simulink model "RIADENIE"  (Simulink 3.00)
settings: Solver=ode45  SolverMode=SingleTasking  StartTime=0.0  StopTime=1.5  FixedStep=0.00001  MaxStep=Auto  RelTol=1e-5
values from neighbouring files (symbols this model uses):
  J = 0.0017    [Data.m]
  Km = Tim/(K3*Tw3)    [Regulatory.m]
  Kmt = Timt/(K2*Tw2)    [Regulatory.m]
  Kpp = T1/(K1*Tw1)    [Regulatory.m]
  kr = Lm/Lr    (= 0.963591022444)    [Data.m]
  Lm = .5796    (= 0.5796)    [Data.m]
  Ls1 = Ls-Lm^2/Lr    (= 0.0430026433915)    [Data.m]
  p = 1    [Data.m]
  R1 = Rs+kr^2*Rr    (= 11.0434783366)    [Data.m]
  T1 = Ls1/R1    (= 0.00389394012293)    [Data.m]
  Tim = (T1*R1)/(Kpp)    [Regulatory.m]
  Timt = Tr    [Regulatory.m]
  Tip = T1    [Regulatory.m]
  Tr = Lr/Rr    (= 0.162567567568)    [Data.m]
  Tvz = 0.001    [Regulatory.m]
undefined symbols (not defined in the file or in its folder): km
libraries: simulink_extras x1

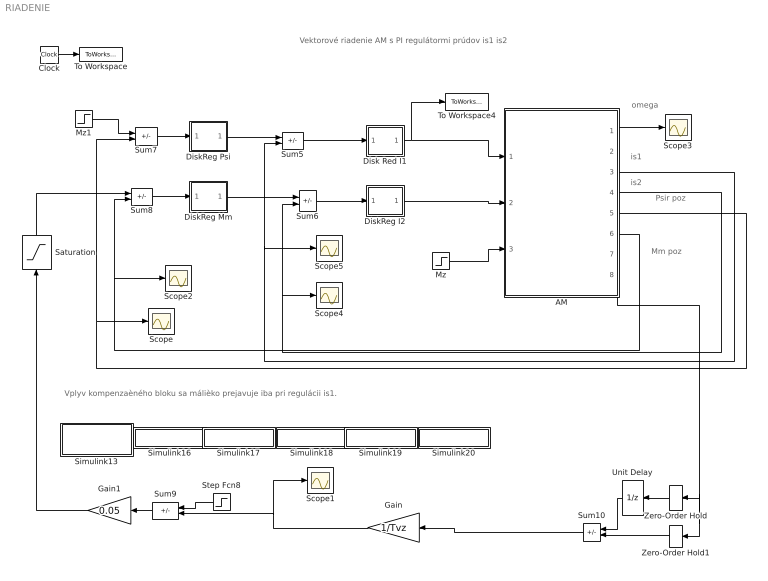
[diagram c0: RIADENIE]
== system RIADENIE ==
  note: omega
  note: Psir poz
  note: Mm poz
  note: is1
  note: is2
  note: Vektorové riadenie AM s PI regulátormi prúdov is1 is2
  note: Vplyv kompenzaèného bloku sa málièko prejavuje iba pri regulácii is1.
  AM : Subsystem
  Clock : Clock
  Disk Red I1 : Subsystem
  DiskReg I2 : Subsystem
  DiskReg Mm : Subsystem
  DiskReg Psi : Subsystem
  Gain : Gain  Orientation=left  Gain=1/Tvz  SaturateOnIntegerOverflow=on
  Gain1 : Gain  Orientation=left  Gain=0.05  SaturateOnIntegerOverflow=on
  Mz : Step  Description=Mz  Time=0  Before=0  After=0  SampleTime=0
  Mz1 : Step  Description=Mz  Time=0  Before=0  After=1  SampleTime=0
  Saturation : Saturate  Orientation=up  UpperLimit=135  LowerLimit=-135
  Scope{,1..5} (6 alike) : Scope
  Simulink13 : Subsystem
  Simulink16 : Subsystem
  Simulink17 : Subsystem
  Simulink18 : Subsystem
  Simulink19 : Subsystem
  Simulink20 : Subsystem
  Step Fcn8 : Step  Orientation=left  Time=0  Before=0  After=100  SampleTime=0
  Sum10 : Sum  Orientation=left  Inputs=-+  SaturateOnIntegerOverflow=on
  Sum{5..8} (4 alike) : Sum  Inputs=+-  SaturateOnIntegerOverflow=on
  Sum9 : Sum  Orientation=left  Inputs=+-  SaturateOnIntegerOverflow=on
  To Workspace : ToWorkspace  VariableName=t  SampleTime=0  SaveFormat=Matrix
  To Workspace4 : ToWorkspace  VariableName=u  SampleTime=0  SaveFormat=Matrix
  Unit Delay : UnitDelay  Orientation=left  X0=0  SampleTime=Tvz
  Zero-Order Hold : ZeroOrderHold  Orientation=left  SampleTime=Tvz
  Zero-Order Hold1 : ZeroOrderHold  Orientation=left  SampleTime=Tvz
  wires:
  Clock/1 -> To Workspace/1
  Sum5/1 -> Disk Red I1/1(In1)
  Disk Red I1/1(Out1) -> AM/1(us1), To Workspace4/1
  Sum6/1 -> DiskReg I2/1(In1)
  DiskReg I2/1(Out1) -> AM/2(us2)
  Sum7/1 -> DiskReg Psi/1(In1)
  Sum8/1 -> DiskReg Mm/1(In1)
  Mz/1 -> AM/3(Mz)
  Step Fcn8/1 -> Sum9/1
  DiskReg Psi/1(Out1) -> Sum5/1
  DiskReg Mm/1(Out1) -> Sum6/1
  Gain1/1 -> Saturation/1
  AM/5(PsirPoz) -> Sum7/2, Scope/1
  AM/4(is2) -> Sum6/2, Scope4/1
  AM/3(is1) -> Sum5/2, Scope5/1
  Saturation/1 -> Sum8/1
  Sum9/1 -> Gain1/1
  Mz1/1 -> Sum7/1
  AM/6(MmPoz) -> Sum8/2, Scope2/1
  Zero-Order Hold1/1 -> Sum10/2
  Unit Delay/1 -> Sum10/1
  Zero-Order Hold/1 -> Unit Delay/1
  AM/1(omega) -> Scope3/1
  Gain/1 -> Scope1/1, Sum9/2
  Sum10/1 -> Gain/1
  AM/8(Theta) -> Zero-Order Hold/1, Zero-Order Hold1/1

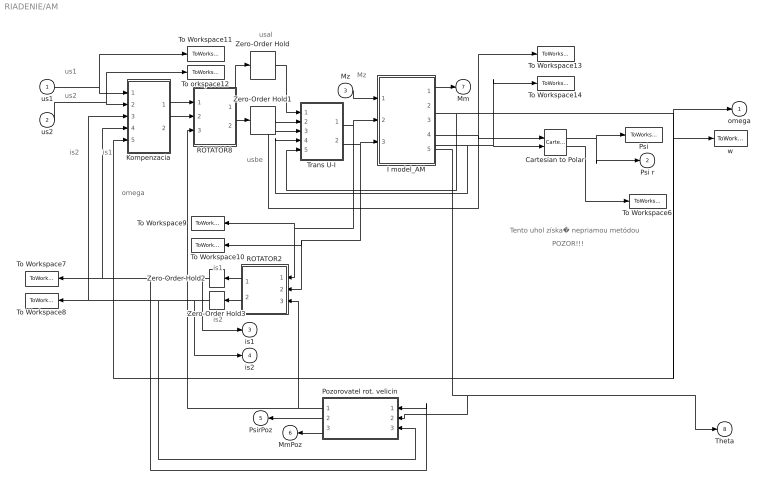
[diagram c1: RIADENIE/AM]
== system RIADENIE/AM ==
  note: is2
  note: is1
  note: omega
  note: us2
  note: us1
  note: Mz
  note: is1
  note: is2
  note: POZOR!!!
  note: Tento uhol získa� nepriamou metódou
  note: usal
  note: usbe
  us1 : Inport  Port=1  PortWidth=-1  SampleTime=-1  DataType=auto
  us2 : Inport  Port=2  PortWidth=-1  SampleTime=-1  DataType=auto
  Mz : Inport  Port=3  PortWidth=-1  SampleTime=-1  DataType=auto
  Cartesian to Polar : simulink_extras/Transformations/Cartesian to Polar
  I model_AM : Subsystem
  Kompenzacia : Subsystem
  Pozorovatel rot. velicin : Subsystem  Orientation=left
  Psi : ToWorkspace  VariableName=Psi  SampleTime=0  SaveFormat=Matrix
  ROTATOR2 : Subsystem  Orientation=left
  ROTATOR8 : Subsystem
  To Workspace10 : ToWorkspace  VariableName=isb  SampleTime=0  SaveFormat=Matrix
  To Workspace11 : ToWorkspace  VariableName=us1  SampleTime=0  SaveFormat=Matrix
  To Workspace13 : ToWorkspace  VariableName=psiral  SampleTime=0  SaveFormat=Matrix
  To Workspace14 : ToWorkspace  VariableName=psirbe  SampleTime=0  SaveFormat=Matrix
  To Workspace6 : ToWorkspace  VariableName=theta  SampleTime=0  SaveFormat=Matrix
  To Workspace7 : ToWorkspace  VariableName=is1  SampleTime=0  SaveFormat=Matrix
  To Workspace8 : ToWorkspace  VariableName=is2  SampleTime=0  SaveFormat=Matrix
  To Workspace9 : ToWorkspace  VariableName=isal  SampleTime=0  SaveFormat=Matrix
  To orkspace12 : ToWorkspace  VariableName=us2  SampleTime=0  SaveFormat=Matrix
  Trans U-I : Subsystem
  Zero-Order Hold : ZeroOrderHold  SampleTime=Tvz
  Zero-Order Hold1 : ZeroOrderHold  SampleTime=Tvz
  Zero-Order Hold2 : ZeroOrderHold  Orientation=left  SampleTime=Tvz
  Zero-Order Hold3 : ZeroOrderHold  Orientation=left  SampleTime=Tvz
  w : ToWorkspace  VariableName=omega  SampleTime=0  SaveFormat=Matrix
  omega : Outport  Port=1  InitialOutput=0
  Psi r : Outport  Port=2  InitialOutput=0
  is1 : Outport  Port=3  InitialOutput=0
  is2 : Outport  Port=4  InitialOutput=0
  PsirPoz : Outport  Orientation=left  Port=5  InitialOutput=0
  MmPoz : Outport  Orientation=left  Port=6  InitialOutput=0
  Mm : Outport  Port=7  InitialOutput=0
  Theta : Outport  Port=8  InitialOutput=0
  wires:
  Kompenzacia/2(Outport2) -> ROTATOR8/2(in_2)
  Kompenzacia/1(Outport1) -> ROTATOR8/1(in_1)
  Trans U-I/2(out_2) -> I model_AM/3(isbe), To Workspace10/1, ROTATOR2/2(in_2)
  Mz/1 -> I model_AM/1(Mz)
  Trans U-I/1(out_1) -> I model_AM/2(isal), To Workspace9/1, ROTATOR2/1(in_1)
  us1/1 -> Kompenzacia/1(in_1), To Workspace11/1
  us2/1 -> Kompenzacia/2(in_2), To orkspace12/1
  Pozorovatel rot. velicin/1(ThetaPoz) -> ROTATOR8/3(in_3), ROTATOR2/3(in_3)
  Pozorovatel rot. velicin/2(PsirPoz) -> PsirPoz/1
  Pozorovatel rot. velicin/3(MmPoz) -> MmPoz/1
  Cartesian to Polar/1 -> Psi/1, Psi r/1
  Cartesian to Polar/2 -> To Workspace6/1
  I model_AM/1(Mm) -> Mm/1
  I model_AM/3(Psir_al) -> Cartesian to Polar/1, To Workspace13/1, Trans U-I/3(in_6)
  I model_AM/4(Psir_be) -> Cartesian to Polar/2, To Workspace14/1, Trans U-I/4(in_4)
  I model_AM/2(omega) -> omega/1, w/1, Kompenzacia/5(in_5), Trans U-I/5(in_8)
  I model_AM/5(Theta) -> Theta/1, Pozorovatel rot. velicin/2(theta)
  ROTATOR8/2(out_2) -> Zero-Order Hold1/1
  Zero-Order Hold1/1 -> Trans U-I/2(in_2)
  ROTATOR8/1(out_1) -> Zero-Order Hold/1
  Zero-Order Hold/1 -> Trans U-I/1(in_1)
  ROTATOR2/1(out_1) -> Zero-Order Hold2/1
  Zero-Order Hold2/1 -> is1/1, Kompenzacia/4(in_6), To Workspace7/1, Pozorovatel rot. velicin/1(Is1)
  ROTATOR2/2(out_2) -> Zero-Order Hold3/1
  Zero-Order Hold3/1 -> is2/1, Kompenzacia/3(in_3), To Workspace8/1, Pozorovatel rot. velicin/3(Is2)

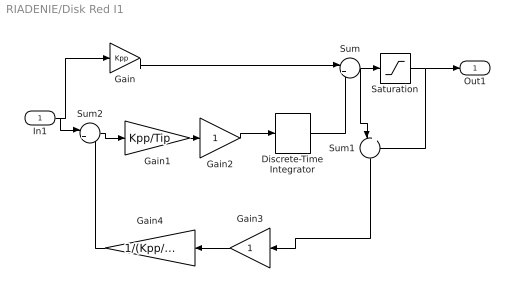
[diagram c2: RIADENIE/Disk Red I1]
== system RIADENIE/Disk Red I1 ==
  In1 : Inport  Port=1  PortWidth=-1  SampleTime=-1  DataType=auto
  Discrete-Time Integrator : DiscreteIntegrator  IntegratorMethod=ForwardEuler  ExternalReset=none  InitialConditionSource=internal  InitialCondition=0  LimitOutput=off  UpperSaturationLimit=inf  LowerSaturationLimit=-inf  ShowSaturationPort=off  ShowStatePort=off  SampleTime=Tvz
  Gain : Gain  Gain=Kpp  SaturateOnIntegerOverflow=on
  Gain1 : Gain  Gain=Kpp/Tip  SaturateOnIntegerOverflow=on
  Gain2 : Gain  Gain=1  SaturateOnIntegerOverflow=on
  Gain3 : Gain  Orientation=left  Gain=1  SaturateOnIntegerOverflow=on
  Gain4 : Gain  Orientation=left  Gain=1/(Kpp/Tip)  SaturateOnIntegerOverflow=on
  Saturation : Saturate  UpperLimit=311  LowerLimit=-311
  Sum : Sum  Inputs=|++  SaturateOnIntegerOverflow=on
  Sum1 : Sum  Orientation=down  Inputs=|+-  SaturateOnIntegerOverflow=on
  Sum2 : Sum  Inputs=|+-  SaturateOnIntegerOverflow=on
  Out1 : Outport  Port=1
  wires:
  Gain3/1 -> Gain4/1
  Saturation/1 -> Sum1/2, Out1/1
  Sum/1 -> Sum1/1, Saturation/1
  Discrete-Time Integrator/1 -> Sum/2
  Gain/1 -> Sum/1
  Gain2/1 -> Discrete-Time Integrator/1
  Gain1/1 -> Gain2/1
  Gain4/1 -> Sum2/2
  In1/1 -> Sum2/1, Gain/1
  Sum2/1 -> Gain1/1
  Sum1/1 -> Gain3/1

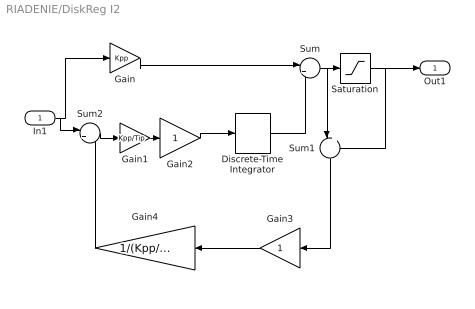
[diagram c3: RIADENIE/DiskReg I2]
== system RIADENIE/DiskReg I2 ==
  In1 : Inport  Port=1  PortWidth=-1  SampleTime=-1  DataType=auto
  Discrete-Time Integrator : DiscreteIntegrator  IntegratorMethod=ForwardEuler  ExternalReset=none  InitialConditionSource=internal  InitialCondition=0  LimitOutput=off  UpperSaturationLimit=inf  LowerSaturationLimit=-inf  ShowSaturationPort=off  ShowStatePort=off  SampleTime=Tvz
  Gain : Gain  Gain=Kpp  SaturateOnIntegerOverflow=on
  Gain1 : Gain  Gain=Kpp/Tip  SaturateOnIntegerOverflow=on
  Gain2 : Gain  Gain=1  SaturateOnIntegerOverflow=on
  Gain3 : Gain  Orientation=left  Gain=1  SaturateOnIntegerOverflow=on
  Gain4 : Gain  Orientation=left  Gain=1/(Kpp/Tip)  SaturateOnIntegerOverflow=on
  Saturation : Saturate  UpperLimit=311  LowerLimit=-311
  Sum : Sum  Inputs=|++  SaturateOnIntegerOverflow=on
  Sum1 : Sum  Orientation=down  Inputs=|+-  SaturateOnIntegerOverflow=on
  Sum2 : Sum  Inputs=|+-  SaturateOnIntegerOverflow=on
  Out1 : Outport  Port=1
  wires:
  Gain1/1 -> Gain2/1
  Gain2/1 -> Discrete-Time Integrator/1
  Gain/1 -> Sum/1
  Discrete-Time Integrator/1 -> Sum/2
  Sum/1 -> Saturation/1, Sum1/1
  Saturation/1 -> Out1/1, Sum1/2
  Sum2/1 -> Gain1/1
  In1/1 -> Gain/1, Sum2/1
  Gain3/1 -> Gain4/1
  Gain4/1 -> Sum2/2
  Sum1/1 -> Gain3/1

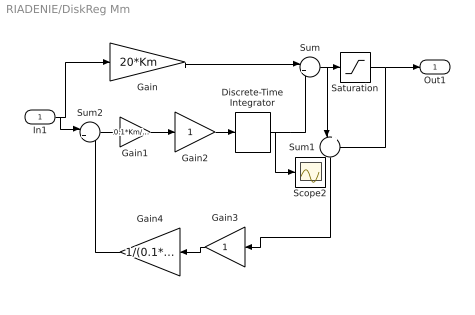
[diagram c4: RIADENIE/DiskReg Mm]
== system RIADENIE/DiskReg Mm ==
  In1 : Inport  Port=1  PortWidth=-1  SampleTime=-1  DataType=auto
  Discrete-Time Integrator : DiscreteIntegrator  IntegratorMethod=ForwardEuler  ExternalReset=none  InitialConditionSource=internal  InitialCondition=0  LimitOutput=off  UpperSaturationLimit=inf  LowerSaturationLimit=-inf  ShowSaturationPort=off  ShowStatePort=off  SampleTime=Tvz
  Gain : Gain  Gain=20*Km  SaturateOnIntegerOverflow=on
  Gain1 : Gain  Gain=0.1*Km/Tim  SaturateOnIntegerOverflow=on
  Gain2 : Gain  Gain=1  SaturateOnIntegerOverflow=on
  Gain3 : Gain  Orientation=left  Gain=1  SaturateOnIntegerOverflow=on
  Gain4 : Gain  Orientation=left  Gain=1/(0.1*Km/Tim)  SaturateOnIntegerOverflow=on
  Saturation : Saturate  UpperLimit=12.28  LowerLimit=-12.28
  Scope2 : Scope
  Sum : Sum  Inputs=|++  SaturateOnIntegerOverflow=on
  Sum1 : Sum  Orientation=down  Inputs=|+-  SaturateOnIntegerOverflow=on
  Sum2 : Sum  Inputs=|+-  SaturateOnIntegerOverflow=on
  Out1 : Outport  Port=1
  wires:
  Gain4/1 -> Sum2/2
  Gain3/1 -> Gain4/1
  In1/1 -> Sum2/1, Gain/1
  Sum2/1 -> Gain1/1
  Saturation/1 -> Sum1/2, Out1/1
  Sum/1 -> Sum1/1, Saturation/1
  Gain/1 -> Sum/1
  Gain2/1 -> Discrete-Time Integrator/1
  Gain1/1 -> Gain2/1
  Sum1/1 -> Gain3/1
  Discrete-Time Integrator/1 -> Sum/2, Scope2/1

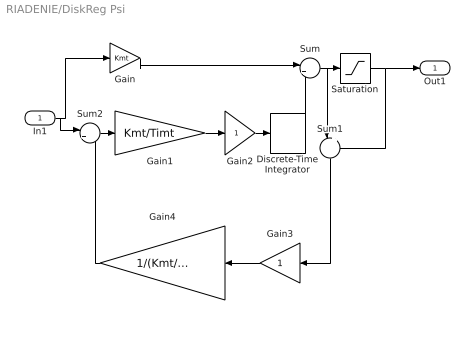
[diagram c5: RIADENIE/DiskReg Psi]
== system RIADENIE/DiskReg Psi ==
  In1 : Inport  Port=1  PortWidth=-1  SampleTime=-1  DataType=auto
  Discrete-Time Integrator : DiscreteIntegrator  IntegratorMethod=ForwardEuler  ExternalReset=none  InitialConditionSource=internal  InitialCondition=0  LimitOutput=off  UpperSaturationLimit=inf  LowerSaturationLimit=-inf  ShowSaturationPort=off  ShowStatePort=off  SampleTime=Tvz
  Gain : Gain  Gain=Kmt  SaturateOnIntegerOverflow=on
  Gain1 : Gain  Gain=Kmt/Timt  SaturateOnIntegerOverflow=on
  Gain2 : Gain  Gain=1  SaturateOnIntegerOverflow=on
  Gain3 : Gain  Orientation=left  Gain=1  SaturateOnIntegerOverflow=on
  Gain4 : Gain  Orientation=left  Gain=1/(Kmt/Timt)  SaturateOnIntegerOverflow=on
  Saturation : Saturate  UpperLimit=12.28  LowerLimit=-12.28
  Sum : Sum  Inputs=|++  SaturateOnIntegerOverflow=on
  Sum1 : Sum  Orientation=down  Inputs=|+-  SaturateOnIntegerOverflow=on
  Sum2 : Sum  Inputs=|+-  SaturateOnIntegerOverflow=on
  Out1 : Outport  Port=1
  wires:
  Gain1/1 -> Gain2/1
  Gain2/1 -> Discrete-Time Integrator/1
  Gain/1 -> Sum/1
  Discrete-Time Integrator/1 -> Sum/2
  Sum/1 -> Saturation/1, Sum1/1
  Saturation/1 -> Out1/1, Sum1/2
  Sum2/1 -> Gain1/1
  In1/1 -> Gain/1, Sum2/1
  Gain3/1 -> Gain4/1
  Gain4/1 -> Sum2/2
  Sum1/1 -> Gain3/1

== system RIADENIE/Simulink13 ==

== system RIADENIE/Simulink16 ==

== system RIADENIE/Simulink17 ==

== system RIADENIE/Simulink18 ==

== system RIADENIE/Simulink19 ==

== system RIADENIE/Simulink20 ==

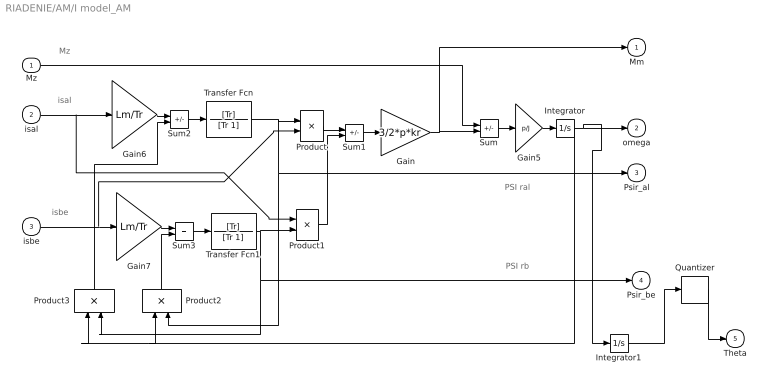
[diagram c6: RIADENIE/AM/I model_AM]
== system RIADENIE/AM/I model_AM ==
  note: isal
  note: PSI ral
  note: isbe
  note: PSI rb
  note: Mz
  Mz : Inport  Port=1  PortWidth=-1  SampleTime=-1  DataType=auto
  isal : Inport  Port=2  PortWidth=-1  SampleTime=-1  DataType=auto
  isbe : Inport  Port=3  PortWidth=-1  SampleTime=-1  DataType=auto
  Gain : Gain  Gain=3/2*p*kr  SaturateOnIntegerOverflow=on
  Gain5 : Gain  Gain=p/J  SaturateOnIntegerOverflow=on
  Gain6 : Gain  Gain=Lm/Tr  SaturateOnIntegerOverflow=on
  Gain7 : Gain  Gain=Lm/Tr  SaturateOnIntegerOverflow=on
  Integrator : Integrator  ExternalReset=none  InitialConditionSource=internal  InitialCondition=0  LimitOutput=off  UpperSaturationLimit=inf  LowerSaturationLimit=-inf  ShowSaturationPort=off  ShowStatePort=off  AbsoluteTolerance=auto
  Integrator1 : Integrator  ExternalReset=none  InitialConditionSource=internal  InitialCondition=0  LimitOutput=off  UpperSaturationLimit=inf  LowerSaturationLimit=-inf  ShowSaturationPort=off  ShowStatePort=off  AbsoluteTolerance=auto
  Product : Product  Inputs=2  SaturateOnIntegerOverflow=on
  Product1 : Product  Inputs=2  SaturateOnIntegerOverflow=on
  Product2 : Product  Orientation=up  Inputs=2  SaturateOnIntegerOverflow=on
  Product3 : Product  Orientation=up  Inputs=2  SaturateOnIntegerOverflow=on
  Quantizer : Quantizer  QuantizationInterval=6.28/4096
  Sum : Sum  Inputs=-+  SaturateOnIntegerOverflow=on
  Sum1 : Sum  Inputs=+-  SaturateOnIntegerOverflow=on
  Sum2 : Sum  Inputs=+-  SaturateOnIntegerOverflow=on
  Sum3 : Sum  Inputs=++  SaturateOnIntegerOverflow=on
  Transfer Fcn : TransferFcn  Numerator=[Tr]  Denominator=[Tr 1]
  Transfer Fcn1 : TransferFcn  Numerator=[Tr]  Denominator=[Tr 1]
  Mm : Outport  Port=1  InitialOutput=0
  omega : Outport  Port=2  InitialOutput=0
  Psir_al : Outport  Port=3  InitialOutput=0
  Psir_be : Outport  Port=4  InitialOutput=0
  Theta : Outport  Port=5  InitialOutput=0
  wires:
  Gain/1 -> Mm/1, Sum/2
  Product1/1 -> Sum1/2
  Mz/1 -> Sum/1
  isbe/1 -> Gain7/1, Product/2
  Product2/1 -> Sum3/2
  Sum3/1 -> Transfer Fcn1/1
  Sum2/1 -> Transfer Fcn/1
  Product/1 -> Sum1/1
  Sum1/1 -> Gain/1
  Sum/1 -> Gain5/1
  Integrator/1 -> Product3/1, Product2/1, omega/1, Integrator1/1
  Transfer Fcn/1 -> Product/1, Product2/2, Psir_al/1
  Gain7/1 -> Sum3/1
  Gain6/1 -> Sum2/1
  Transfer Fcn1/1 -> Product1/2, Product3/2, Psir_be/1
  Product3/1 -> Sum2/2
  isal/1 -> Gain6/1, Product1/1
  Gain5/1 -> Integrator/1
  Integrator1/1 -> Quantizer/1
  Quantizer/1 -> Theta/1

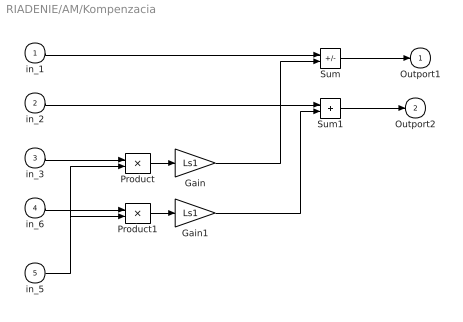
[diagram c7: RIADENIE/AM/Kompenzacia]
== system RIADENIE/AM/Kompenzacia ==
  in_1 : Inport  Port=1  PortWidth=-1  SampleTime=-1  DataType=auto
  in_2 : Inport  Port=2  PortWidth=-1  SampleTime=-1  DataType=auto
  in_3 : Inport  Port=3  PortWidth=-1  SampleTime=-1  DataType=auto
  in_6 : Inport  Port=4  PortWidth=-1  SampleTime=-1  DataType=auto
  in_5 : Inport  Port=5  PortWidth=-1  SampleTime=-1  DataType=auto
  Gain : Gain  Gain=Ls1  SaturateOnIntegerOverflow=on
  Gain1 : Gain  Gain=Ls1  SaturateOnIntegerOverflow=on
  Product : Product  Inputs=2  SaturateOnIntegerOverflow=on
  Product1 : Product  Inputs=2  SaturateOnIntegerOverflow=on
  Sum : Sum  Inputs=+-  SaturateOnIntegerOverflow=on
  Sum1 : Sum  Inputs=++  SaturateOnIntegerOverflow=on
  Outport1 : Outport  Port=1  InitialOutput=0
  Outport2 : Outport  Port=2  InitialOutput=0
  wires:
  Sum1/1 -> Outport2/1
  in_2/1 -> Sum1/1
  Gain1/1 -> Sum1/2
  Product1/1 -> Gain1/1
  in_5/1 -> Product/2, Product1/2
  in_6/1 -> Product1/1
  Sum/1 -> Outport1/1
  Gain/1 -> Sum/2
  in_1/1 -> Sum/1
  Product/1 -> Gain/1
  in_3/1 -> Product/1

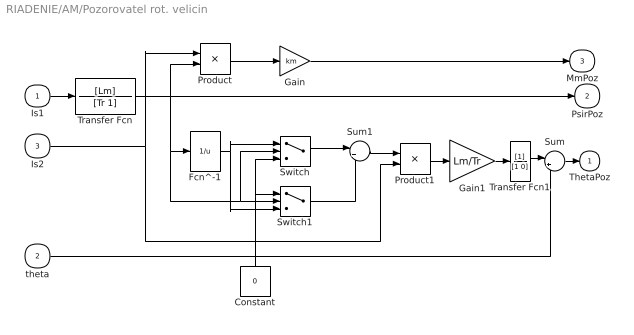
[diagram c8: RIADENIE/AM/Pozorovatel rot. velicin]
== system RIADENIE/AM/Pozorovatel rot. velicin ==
  Is1 : Inport  Port=1  PortWidth=-1  SampleTime=-1  DataType=auto
  theta : Inport  Port=2  PortWidth=-1  SampleTime=-1  DataType=auto
  Is2 : Inport  Port=3  PortWidth=-1  SampleTime=-1  DataType=auto
  Constant : Constant  Orientation=up  Value=0
  Fcn^-1 : Fcn  Expr=1/u
  Gain : Gain  Gain=km  SaturateOnIntegerOverflow=on
  Gain1 : Gain  Gain=Lm/Tr  SaturateOnIntegerOverflow=on
  Product : Product  Inputs=2  SaturateOnIntegerOverflow=on
  Product1 : Product  Inputs=2  SaturateOnIntegerOverflow=on
  Sum : Sum  Inputs=|++  SaturateOnIntegerOverflow=on
  Sum1 : Sum  Inputs=|++  SaturateOnIntegerOverflow=on
  Switch : Switch  Threshold=0.001
  Switch1 : Switch  Threshold=-0.001
  Transfer Fcn : TransferFcn  Numerator=[Lm]  Denominator=[Tr 1]
  Transfer Fcn1 : TransferFcn  Numerator=[1]  Denominator=[1 0]
  ThetaPoz : Outport  Port=1
  PsirPoz : Outport  Port=2
  MmPoz : Outport  Port=3
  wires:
  Is1/1 -> Transfer Fcn/1
  Transfer Fcn/1 -> PsirPoz/1, Product/2, Fcn^-1/1, Switch1/2, Switch/2
  Gain/1 -> MmPoz/1
  Product/1 -> Gain/1
  Is2/1 -> Product/1, Product1/2
  Fcn^-1/1 -> Switch/1, Switch1/3
  Transfer Fcn1/1 -> Sum/1
  theta/1 -> Sum/2
  Sum/1 -> ThetaPoz/1
  Gain1/1 -> Transfer Fcn1/1
  Product1/1 -> Gain1/1
  Sum1/1 -> Product1/1
  Switch1/1 -> Sum1/2
  Switch/1 -> Sum1/1
  Constant/1 -> Switch/3, Switch1/1

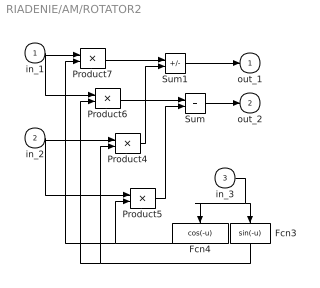
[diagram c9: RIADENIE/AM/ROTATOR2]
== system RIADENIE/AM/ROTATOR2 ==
  in_1 : Inport  Port=1  PortWidth=-1  SampleTime=-1  DataType=auto
  in_2 : Inport  Port=2  PortWidth=-1  SampleTime=-1  DataType=auto
  in_3 : Inport  Port=3  PortWidth=-1  SampleTime=-1  DataType=auto
  Fcn3 : Fcn  Orientation=down  Expr=sin(-u)
  Fcn4 : Fcn  Orientation=down  Expr=cos(-u)
  Product{4..7} (4 alike) : Product  Inputs=2  SaturateOnIntegerOverflow=on
  Sum : Sum  Inputs=++  SaturateOnIntegerOverflow=on
  Sum1 : Sum  Inputs=+-  SaturateOnIntegerOverflow=on
  out_1 : Outport  Port=1  InitialOutput=0
  out_2 : Outport  Port=2  InitialOutput=0
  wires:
  in_3/1 -> Fcn3/1, Fcn4/1
  in_2/1 -> Product5/1, Product4/1
  Sum/1 -> out_2/1
  Sum1/1 -> out_1/1
  in_1/1 -> Product6/1, Product7/1
  Product4/1 -> Sum1/2
  Product7/1 -> Sum1/1
  Fcn3/1 -> Product4/2, Product6/2
  Product6/1 -> Sum/1
  Product5/1 -> Sum/2
  Fcn4/1 -> Product7/2, Product5/2

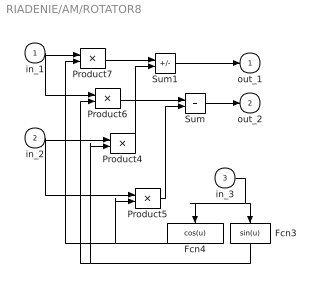
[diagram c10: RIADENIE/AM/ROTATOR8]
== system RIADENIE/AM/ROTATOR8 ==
  in_1 : Inport  Port=1  PortWidth=-1  SampleTime=-1  DataType=auto
  in_2 : Inport  Port=2  PortWidth=-1  SampleTime=-1  DataType=auto
  in_3 : Inport  Port=3  PortWidth=-1  SampleTime=-1  DataType=auto
  Fcn3 : Fcn  Orientation=down  Expr=sin(u)
  Fcn4 : Fcn  Orientation=down  Expr=cos(u)
  Product{4..7} (4 alike) : Product  Inputs=2  SaturateOnIntegerOverflow=on
  Sum : Sum  Inputs=++  SaturateOnIntegerOverflow=on
  Sum1 : Sum  Inputs=+-  SaturateOnIntegerOverflow=on
  out_1 : Outport  Port=1  InitialOutput=0
  out_2 : Outport  Port=2  InitialOutput=0
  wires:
  Fcn4/1 -> Product7/2, Product5/2
  Product5/1 -> Sum/2
  Product6/1 -> Sum/1
  Fcn3/1 -> Product4/2, Product6/2
  Product7/1 -> Sum1/1
  Product4/1 -> Sum1/2
  in_1/1 -> Product7/1, Product6/1
  Sum1/1 -> out_1/1
  Sum/1 -> out_2/1
  in_2/1 -> Product4/1, Product5/1
  in_3/1 -> Fcn3/1, Fcn4/1

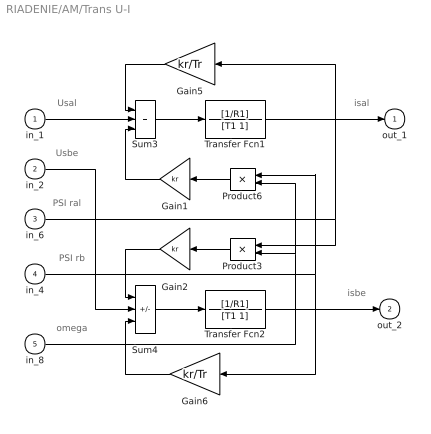
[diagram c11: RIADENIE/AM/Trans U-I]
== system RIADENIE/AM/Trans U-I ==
  note: PSI rb
  note: PSI ral
  note: omega
  note: Usal
  note: Usbe
  note: isal
  note: isbe
  in_1 : Inport  Port=1  PortWidth=-1  SampleTime=-1  DataType=auto
  in_2 : Inport  Port=2  PortWidth=-1  SampleTime=-1  DataType=auto
  in_6 : Inport  Port=3  PortWidth=-1  SampleTime=-1  DataType=auto
  in_4 : Inport  Port=4  PortWidth=-1  SampleTime=-1  DataType=auto
  in_8 : Inport  Port=5  PortWidth=-1  SampleTime=-1  DataType=auto
  Gain1 : Gain  Orientation=left  Gain=kr  SaturateOnIntegerOverflow=on
  Gain2 : Gain  Orientation=left  Gain=kr  SaturateOnIntegerOverflow=on
  Gain5 : Gain  Orientation=left  Gain=kr/Tr  SaturateOnIntegerOverflow=on
  Gain6 : Gain  Orientation=left  Gain=kr/Tr  SaturateOnIntegerOverflow=on
  Product3 : Product  Orientation=left  Inputs=2  SaturateOnIntegerOverflow=on
  Product6 : Product  Orientation=left  Inputs=2  SaturateOnIntegerOverflow=on
  Sum3 : Sum  Inputs=+++  SaturateOnIntegerOverflow=on
  Sum4 : Sum  Inputs=-++  SaturateOnIntegerOverflow=on
  Transfer Fcn1 : TransferFcn  Numerator=[1/R1]  Denominator=[T1 1]
  Transfer Fcn2 : TransferFcn  Numerator=[1/R1]  Denominator=[T1 1]
  out_1 : Outport  Port=1  InitialOutput=0
  out_2 : Outport  Port=2  InitialOutput=0
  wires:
  in_2/1 -> Sum4/2
  Gain1/1 -> Sum3/3
  Gain2/1 -> Sum4/1
  Transfer Fcn2/1 -> out_2/1
  Transfer Fcn1/1 -> out_1/1
  Sum3/1 -> Transfer Fcn1/1
  Sum4/1 -> Transfer Fcn2/1
  Gain6/1 -> Sum4/3
  Gain5/1 -> Sum3/1
  in_1/1 -> Sum3/2
  Product6/1 -> Gain1/1
  Product3/1 -> Gain2/1
  in_8/1 -> Product6/2, Product3/2
  in_6/1 -> Product3/1, Gain5/1
  in_4/1 -> Gain6/1, Product6/1
